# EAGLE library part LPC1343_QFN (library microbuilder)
LPC1343 72 MHz 32-bit ARM Cortex-M3 based microcontroller featuring a high level of integration and low power consumption. 32 kB Flash, 8 kB SRAM, USB Device MarcVl - Datasheet available on www.nxp.com
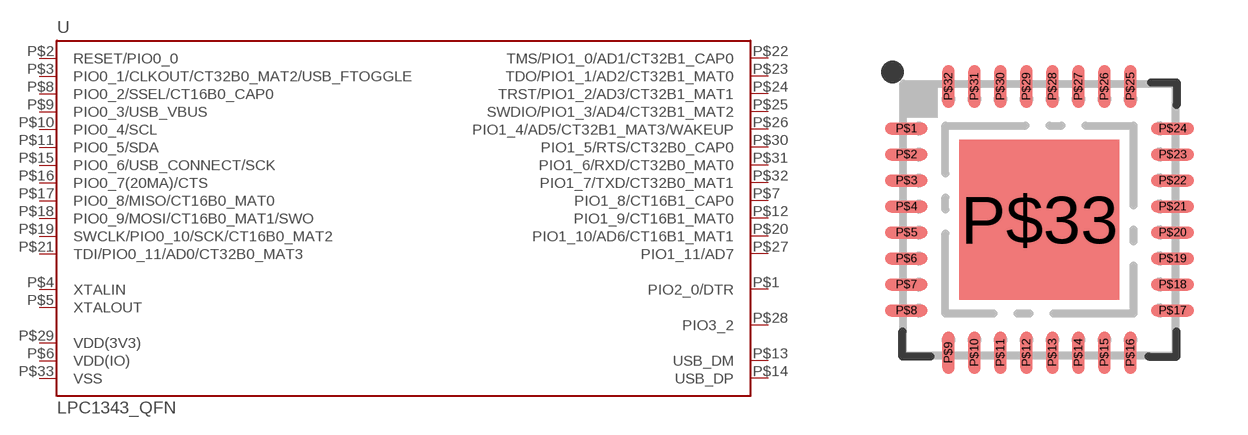
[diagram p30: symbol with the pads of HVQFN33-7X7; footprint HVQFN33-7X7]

Designator prefix U

## LPC1343_QFN (DIGIKEY#: 568-4944-ND; MANF: NXP; MANF#: LPC1343FHN33,551)  [HVQFN33-7X7]
P$1  PIO2_0/DTR
P$2  RESET/PIO0_0
P$3  PIO0_1/CLKOUT/CT32B0_MAT2/USB_FTOGGLE
P$4  XTALIN  in
P$5  XTALOUT  out
P$6  VDD(IO)  pwr
P$7  PIO1_8/CT16B1_CAP0
P$8  PIO0_2/SSEL/CT16B0_CAP0
P$9  PIO0_3/USB_VBUS
P$10  PIO0_4/SCL
P$11  PIO0_5/SDA
P$12  PIO1_9/CT16B1_MAT0
P$13  USB_DM
P$14  USB_DP
P$15  PIO0_6/USB_CONNECT/SCK
P$16  PIO0_7(20MA)/CTS
P$17  PIO0_8/MISO/CT16B0_MAT0
P$18  PIO0_9/MOSI/CT16B0_MAT1/SWO
P$19  SWCLK/PIO0_10/SCK/CT16B0_MAT2
P$20  PIO1_10/AD6/CT16B1_MAT1
P$21  TDI/PIO0_11/AD0/CT32B0_MAT3
P$22  TMS/PIO1_0/AD1/CT32B1_CAP0
P$23  TDO/PIO1_1/AD2/CT32B1_MAT0
P$24  TRST/PIO1_2/AD3/CT32B1_MAT1
P$25  SWDIO/PIO1_3/AD4/CT32B1_MAT2
P$26  PIO1_4/AD5/CT32B1_MAT3/WAKEUP
P$27  PIO1_11/AD7
P$28  PIO3_2
P$29  VDD(3V3)  pwr
P$30  PIO1_5/RTS/CT32B0_CAP0
P$31  PIO1_6/RXD/CT32B0_MAT0
P$32  PIO1_7/TXD/CT32B0_MAT1
P$33  VSS  pwr

## Footprint HVQFN33-7X7 (pad centres in mm)
HVQFN33 Plastic thermal enhanced very thin quad flat package; 33 terminals; body 7x7x0.85 mm; Thermal pad intentionally smaller than actual pad size to avoid bridges
smd 1.067 x 0.3: P$1 -3.327,2.275; P$2 -3.327,1.625; P$3 -3.327,0.975; P$4 -3.327,0.325; P$5 -3.327,-0.325; P$6 -3.327,-0.975; P$7 -3.327,-1.625; P$8 -3.327,-2.275; P$17 3.327,-2.275; P$18 3.327,-1.625; P$19 3.327,-0.975; P$20 3.327,-0.325; P$21 3.327,0.325; P$22 3.327,0.975; P$23 3.327,1.625; P$24 3.327,2.275
smd 0.3 x 1.067: P$9 -2.275,-3.327; P$10 -1.625,-3.327; P$11 -0.975,-3.327; P$12 -0.325,-3.327; P$13 0.325,-3.327; P$14 0.975,-3.327; P$15 1.625,-3.327; P$16 2.275,-3.327; P$25 2.275,3.327; P$26 1.625,3.327; P$27 0.975,3.327; P$28 0.325,3.327; P$29 -0.325,3.327; P$30 -0.975,3.327; P$31 -1.625,3.327; P$32 -2.275,3.327
smd 4 x 4: P$33 0,0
